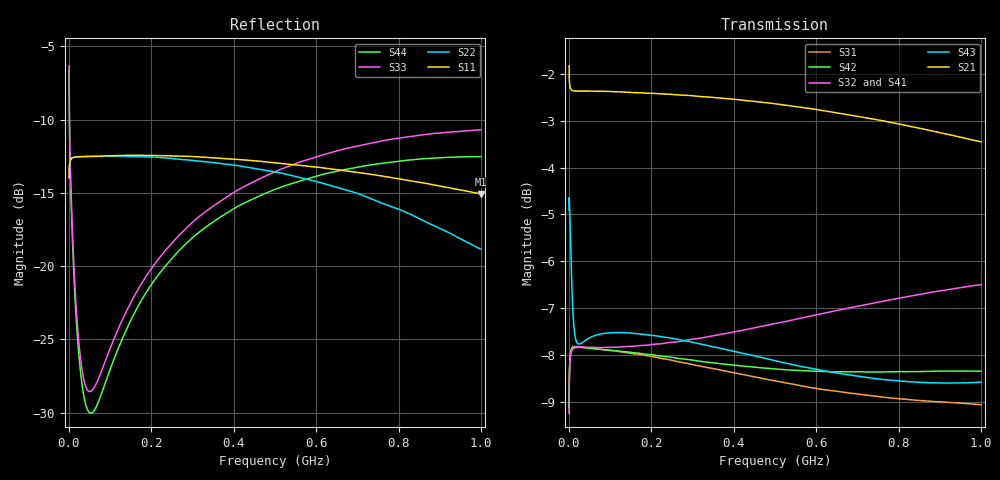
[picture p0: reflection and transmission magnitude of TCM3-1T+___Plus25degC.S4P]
!MINI CIRCUITS LABORATORY
!S-PARAMETER
!MODEL:TCM3-1T+
!RUN/LOT/DATE CODE:MB27010/0641
!FIXTURE USED:90-2-20-199
!CONNECTION:PORT1-PIN6,PORT2-PIN4,PORT3-PIN1,PORT4-PIN3
!NETWORK ANALYZER: Agilent Technologies,E5071C,MY46100909,A.08.01
!Agilent Technologies,E5071C,MY46100909,A.08.01
!Date: Thu Dec 20 10:32:13 2007
# Hz S dB R 50
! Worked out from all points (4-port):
!   929 points, 300 kHz to 1 GHz, reference 50 ohm
!   strongest paths, dB at 300 kHz, 127 MHz, 243 MHz, 436 MHz, 1 GHz:
!     S21: -1.8, -2.4, -2.4, -2.6, -3.5
!     S43: -4.9, -7.5, -7.6, -8.0, -8.6
!     S32: -9.2, -7.8, -7.7, -7.4, -6.5
!     S41: -9.1, -7.8, -7.8, -7.5, -6.7
!     S42: -9.1, -7.9, -8.0, -8.2, -8.3
!     S31: -9.2, -7.9, -8.1, -8.4, -9.1
!   lowest |S11| = -15.1 dB at 1 GHz (marker M1), VSWR 1.43, Z = 48 - j17.4 ohm
!   |S11| at or under -10 dB: start of sweep to end of sweep
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300000  -13.98 20.7  -1.84 -4.8  -9.29 20.1  -9.16 -160.2
        -1.84 -4.8  -13.96 20.3  -9.31 -159.8  -9.17 19.9
        -9.22 20.6  -9.24 -159.2  -6.35 148.8  -4.91 -163.7
        -9.09 -159.6  -9.11 20.5  -4.92 -163.6  -6.62 146.9
5000000  -12.68 2.6  -2.34 -1.2  -7.95 2.7  -7.87 -177.7
         -2.34 -1.2  -12.67 2.6  -7.93 -177.4  -7.87 2.4
         -7.94 2.7  -7.93 -177.5  -14.85 117.9  -5.98 169.8
         -7.86 -177.7  -7.88 2.4  -5.98 169.8  -15.46 115.3
1.8e7  -12.55 -0.1  -2.38 -1.4  -7.84 0.3  -7.80 179.4
       -2.37 -1.3  -12.55 -0.0  -7.82 179.6  -7.81 0.2
       -7.84 0.3  -7.82 179.6  -23.06 71.4  -7.71 173.4
       -7.80 179.4  -7.81 0.2  -7.70 173.4  -23.82 65.4
5.2e7  -12.51 -2.6  -2.38 -3.1  -7.86 -1.2  -7.84 176.8
       -2.37 -3.1  -12.51 -2.4  -7.83 176.8  -7.85 -1.0
       -7.85 -1.2  -7.83 176.7  -28.56 61.1  -7.62 175.3
       -7.84 176.9  -7.85 -1.0  -7.62 175.2  -30.05 55.1
1.91e8  -12.44 -11.1  -2.42 -10.8  -8.01 -4.4  -7.80 168.8
        -2.42 -10.8  -12.54 -10.6  -7.78 168.0  -7.98 -3.3
        -8.01 -4.4  -7.78 167.9  -20.53 69.1  -7.57 164.0
        -7.81 168.8  -7.98 -3.3  -7.57 164.0  -21.63 70.0
3.64e8  -12.64 -23.4  -2.52 -20.3  -8.30 -7.0  -7.61 158.6
        -2.52 -20.3  -12.98 -22.6  -7.56 156.9  -8.16 -5.1
        -8.31 -7.0  -7.56 156.9  -15.64 56.3  -7.84 150.4
        -7.61 158.6  -8.17 -5.1  -7.84 150.4  -16.71 58.8
1e9  -15.07 -86.5  -3.46 -55.8  -9.07 -10.4  -6.75 116.3
     -3.45 -55.8  -18.84 -93.8  -6.49 110.9  -8.36 -9.6
     -9.05 -10.4  -6.49 110.9  -10.70 6.4  -8.57 113.0
     -6.75 116.4  -8.34 -9.6  -8.57 113.0  -12.53 18.5
